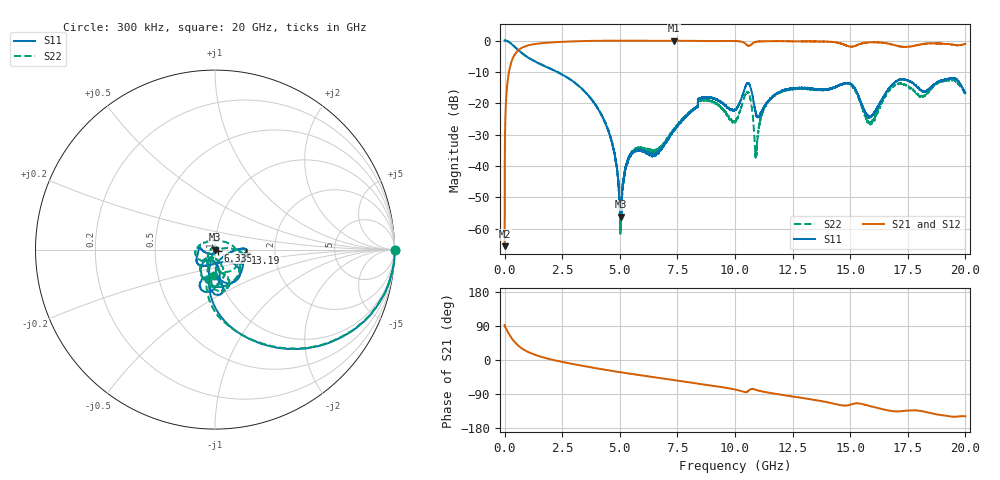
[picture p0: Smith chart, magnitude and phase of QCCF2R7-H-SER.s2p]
!QCCF2R7
!Johanson Technology Inc.
!www.johansontechnology.com
!Test Board Conditions:
!Substrate Type  RO4350B
!Substrate Thickness  10 mil
!Substrate Dk  3.66
!TL Type: GCPW
!TL Trace Width  21 mil
!TL Gap  20 mil
!Electrode orientation  Horizontal
!DUT TOPOLOGY	SERIES
!Mounting Pad LxW  16x21 mil
# MHz S  dB  R 50
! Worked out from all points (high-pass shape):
!   20001 points, 300 kHz to 20 GHz, reference 50 ohm
!   highest |S21| = -0.04 dB at 7.343 GHz (marker M1); lowest = -65.6 dB at 300 kHz (marker M2)
!   |S21| within 3 dB of the highest: 603.3 MHz to end of sweep
!   lowest |S11| = -56.2 dB at 5.047 GHz (marker M3), VSWR 1.00, Z = 50.2 + j0.0187 ohm
!   |S11| at or under -10 dB: 2.281 GHz to end of sweep
!   |S22| runs from -61.6 to 0.0 dB; largest |S21 - S12| = 0.02
!   S11 on the Smith chart (normalised r, x): 300 kHz: open; 6.335 GHz: 1.03, -0.01; 13.19 GHz: 1.41, -0.05; 20 GHz: 0.94, -0.28
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0.3  0.03 -0.0  -65.57 92.5  -65.82 86.6  0.02 -0.0
123.298  -0.19 -13.8  -13.43 76.0  -13.45 76.0  -0.20 -13.8
418.294  -1.86 -40.8  -4.72 48.7  -4.71 48.8  -1.88 -40.7
1300.28  -6.62 -75.7  -1.12 14.1  -1.11 13.9  -6.56 -75.5
3334.25  -15.21 -101.7  -0.18 -14.8  -0.18 -14.7  -15.25 -106.0
4548.232  -29.68 -114.5  -0.05 -27.7  -0.05 -27.7  -29.59 -112.8
5047.224  -56.16 6.9  -0.06 -32.5  -0.05 -32.5  -57.54 -3.6
5452.218  -36.76 38.1  -0.06 -36.3  -0.06 -36.3  -36.46 65.6
6335.205  -36.02 -21.5  -0.07 -44.1  -0.07 -44.2  -35.15 110.2
6667.2  -36.01 -71.0  -0.06 -47.2  -0.07 -47.1  -34.92 147.8
7343.19  -28.92 -138.0  -0.04 -53.2  -0.05 -53.1  -28.47 -150.4
8525.172  -18.44 -148.8  -0.12 -63.7  -0.13 -63.6  -19.13 -157.6
10000.15  -22.05 -67.4  -0.15 -78.0  -0.17 -77.7  -25.99 79.3
10564.14  -13.57 -59.8  -1.62 -82.4  -1.58 -82.1  -16.46 -49.9
10924.14  -23.77 -67.7  -0.39 -79.1  -0.37 -79.0  -35.76 -22.5
11580.13  -18.25 -0.8  -0.22 -87.4  -0.18 -87.7  -18.34 -0.6
13194.1  -15.30 -5.5  -0.26 -102.9  -0.29 -103.1  -15.36 -21.7
13334.1  -15.46 -7.1  -0.29 -104.1  -0.31 -104.2  -15.58 -22.7
14976.08  -13.60 -85.0  -1.92 -118.6  -1.86 -118.6  -13.89 -91.9
15853.06  -24.32 -107.4  -0.56 -121.4  -0.59 -121.6  -26.19 -107.7
16667.05  -15.43 -82.0  -0.99 -133.3  -0.99 -133.9  -16.05 -71.4
20000  -16.73 -94.0  -1.06 -148.6  -0.95 -148.0  -16.82 -93.2
